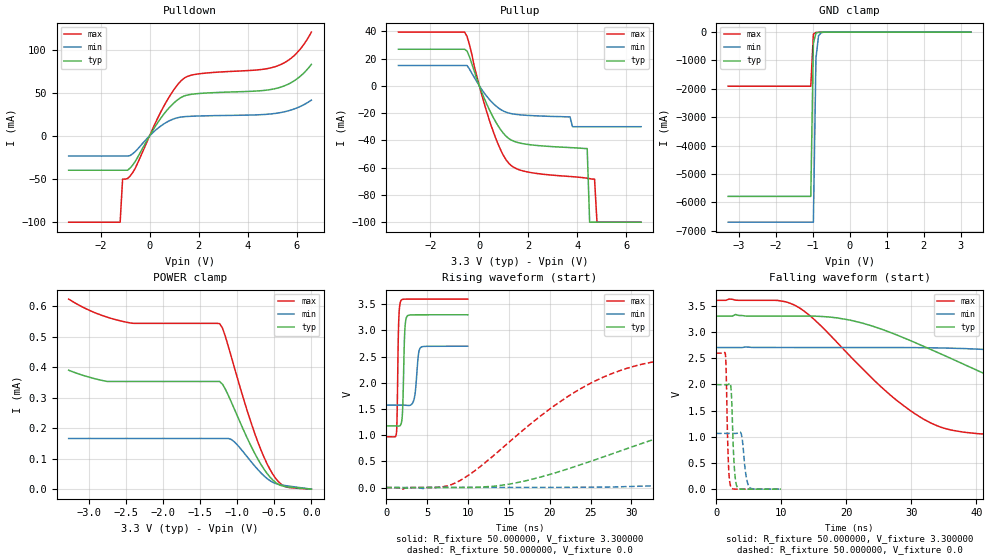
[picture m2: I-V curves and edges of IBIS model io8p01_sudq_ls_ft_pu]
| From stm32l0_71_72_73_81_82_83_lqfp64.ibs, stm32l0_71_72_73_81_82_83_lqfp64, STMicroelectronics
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|   Model io8p01_sudq_ls_ft_pu
[Model]  io8p01_sudq_ls_ft_pu
Model_type I/O
Polarity   Non-Inverting
Enable   Active-Low
Vinl =   0.990000V
Vinh =   2.310000V
Vmeas =  1.650000V
Cref =   50.000000pF
Rref =   100.000000M
Vref =   0.0V
C_comp   2.343000pF   2.309800pF   2.393900pF
[Temperature Range]   25.000000   0.125000k   -40.000000
[Pullup Reference]   3.300000V   2.700000V   3.600000V
[Pulldown Reference]   0.0V   0.0V   0.0V
[POWER Clamp Reference]   3.300000V   2.700000V   3.600000V
[GND Clamp Reference]   0.0V   0.0V   0.0V
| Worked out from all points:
|   slope of the pulldown table from 0 to 0.495 V, typ, clamps not added: 22.6 ohm
|   slope of the pullup table from 0 to 0.495 V, typ, clamps not added: 23.9 ohm
|   GND clamp passes 1 mA (typ) near -0.64 V on its own axis
|   rising waveform, R_fixture 50.000000, V_fixture 3.300000: 20-80 % time 207ps typ, 362ps min, 164ps max; typ from 1.18 V to 3.3 V
|   rising waveform, R_fixture 50.000000, V_fixture 0.0: 20-80 % time 27.2ns typ, 59.9ns min, 13.7ns max; typ from 0.001 V to 1.99 V
|   falling waveform, R_fixture 50.000000, V_fixture 3.300000: 20-80 % time 24.4ns typ, 53.6ns min, 13.4ns max; typ from 3.3 V to 1.18 V
|   falling waveform, R_fixture 50.000000, V_fixture 0.0: 20-80 % time 385ps typ, 557ps min, 306ps max; typ from 1.99 V to 0.001 V
[Pulldown]
|Voltage   I(typ)   I(min)   I(max)
-3.3V     -39.8mA    -23.38mA   -100mA
-1.2V     -39.8mA    -23.38mA   -100mA
-1.1V     -39.8mA    -23.38mA   -50.11mA
-900mV    -39.8mA    -23.38mA   -49.43mA
-700mV    -34.25mA   -21mA      -43.13mA
600mV     25.84mA    14.18mA    35.34mA
1V        38.32mA    19.82mA    53.81mA
1.4V      46.09mA    22.19mA    66.63mA
2V        49.05mA    23.02mA    71.83mA
5.2V      55.23mA    26.32mA    80.92mA
6V        65.77mA    32.26mA    95.84mA
6.6V      82.81mA    41.44mA    120.2mA
[Pullup]
|Voltage   I(typ)   I(min)   I(max)
-3.3V     26.78mA    14.88mA    39.37mA
-600mV    26.78mA    14.88mA    39.37mA
500mV     -20.88mA   -11.78mA   -30.07mA
1.2V      -38.62mA   -19.99mA   -56.79mA
1.9V      -42.8mA    -21.61mA   -62.92mA
3.7V      -45.29mA   -22.8mA    -66.51mA
3.8V      -45.39mA   -30mA      -66.64mA
4.4V      -46.01mA   -30mA      -67.77mA
4.5V      -100mA     -30mA      -68.06mA
4.7V      -100mA     -30mA      -68.41mA
4.8V      -100mA     -30mA      -100mA
6.6V      -100mA     -30mA      -100mA
[GND_clamp]
|Voltage   I(typ)   I(min)   I(max)
-3.3V     -5.787A    -6.696A    -1.906A
-1.06V    -5.787A    -6.696A    -1.906A
-990mV    -393.4mA   -6.696A    -70.75mA
-920mV    -33.02mA   -919.4mA   -10.9mA
-850mV    -6.829mA   -131.3mA   -6.521mA
-780mV    -3.478mA   -21.06mA   -4.208mA
3.28V     0A         0A         0A
[POWER_clamp]
|Voltage   I(typ)   I(min)   I(max)
-3.28V    390.5uA    166.4uA    624.1uA
-2.76V    353.6uA    166.4uA    564.6uA
-2.44V    353.6uA    166.4uA    545.3uA
-1.24V    353.6uA    166.4uA    543.5uA
-1.2V     344.2uA    166.4uA    528.2uA
-1.16V    327.1uA    166.4uA    499.5uA
-1.04V    262.6uA    155.2uA    398.8uA
-760mV    115.1uA    74.4uA     179.3uA
-560mV    39.86uA    27.94uA    65.07uA
-440mV    15uA       15.53uA    23.15uA
-360mV    8.745uA    12.05uA    9.089uA
0V        0A         0A         0A
[Ramp]
| variable   typ   min   max
dV/dt_r  1.19492/27.12827n   0.63569/59.89298n   1.55547/13.62920n
dV/dt_f  1.27326/24.42227n   0.66960/53.54375n   1.57748/13.41274n
R_load = 50.000000
[Rising Waveform]
R_fixture= 50.000000
V_fixture= 3.300000
V_fixture_min= 2.700000
V_fixture_max= 3.600000
|time   V(typ)   V(min)   V(max)
0s        1.178V     1.575V     970.9mV
1.241ns   1.177V     1.575V     1.04V
1.522ns   1.174V     1.575V     3.174V
1.802ns   1.214V     1.575V     3.572V
2.002ns   1.498V     1.575V     3.594V
2.262ns   2.978V     1.574V     3.598V
2.543ns   3.272V     1.57V      3.599V
3.423ns   3.299V     1.703V     3.6V
4.244ns   3.3V       2.68V      3.6V
9.97ns    3.3V       2.7V       3.6V
[Rising Waveform]
R_fixture= 50.000000
V_fixture= 0.0
V_fixture_min= 0.0
V_fixture_max= 0.0
|time   V(typ)   V(min)   V(max)
0s        1.061mV    1.816mV    656.8uV
8.008ns   3.234mV    4.296mV    60.48mV
15.52ns   79.67mV    4.301mV    934.4mV
25.03ns   502.9mV    8.321mV    1.995V
31.03ns   829.9mV    26.85mV    2.348V
39.04ns   1.217V     74.82mV    2.517V
58.06ns   1.756V     284.6mV    2.584V
82.58ns   1.948V     595mV      2.593V
140.6ns   1.992V     975.4mV    2.593V
249.2ns   1.993V     1.064V     2.593V
[Falling Waveform]
R_fixture= 50.000000
V_fixture= 3.300000
V_fixture_min= 2.700000
V_fixture_max= 3.600000
|time   V(typ)   V(min)   V(max)
0s        3.3V       2.7V       3.6V
12.01ns   3.3V       2.7V       3.512V
20.52ns   3.224V     2.7V       2.545V
29.53ns   2.849V     2.699V     1.525V
34.53ns   2.578V     2.692V     1.182V
40.04ns   2.269V     2.67V      1.06V
57.06ns   1.485V     2.525V     989.5mV
77.58ns   1.262V     2.246V     975.1mV
126.6ns   1.188V     1.734V     971mV
249.2ns   1.178V     1.575V     970.9mV
[Falling Waveform]
R_fixture= 50.000000
V_fixture= 0.0
V_fixture_min= 0.0
V_fixture_max= 0.0
|time   V(typ)   V(min)   V(max)
0s        1.993V     1.064V     2.593V
1.441ns   1.993V     1.064V     2.564V
1.902ns   1.997V     1.064V     496.3mV
2.302ns   1.916V     1.064V     40.47mV
2.763ns   509.2mV    1.064V     2.82mV
3.183ns   60.01mV    1.066V     656.2uV
3.924ns   2.054mV    1.026V     611.9uV
4.605ns   1.068mV    262.2mV    615uV
5.125ns   1.056mV    35.94mV    618.8uV
9.97ns    1.061mV    1.816mV    656.8uV
